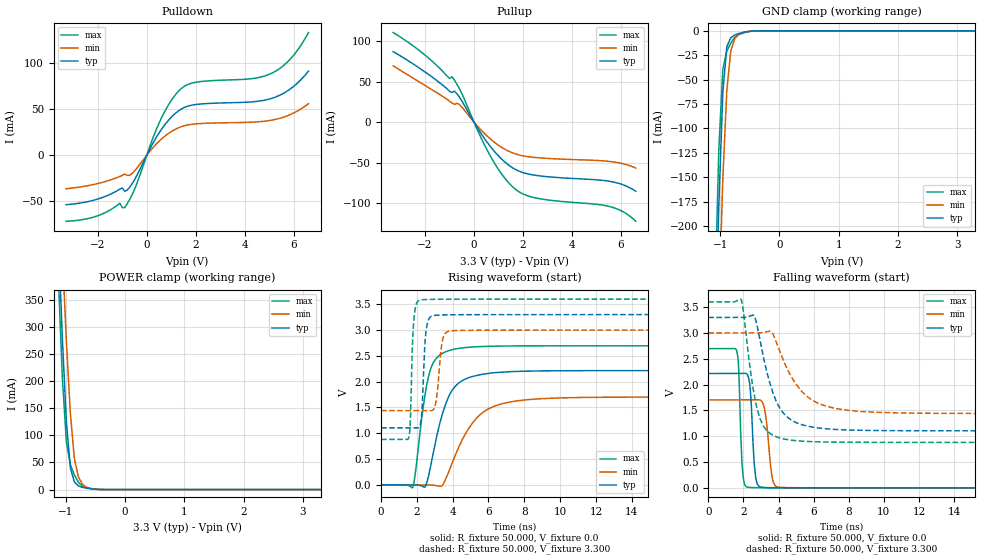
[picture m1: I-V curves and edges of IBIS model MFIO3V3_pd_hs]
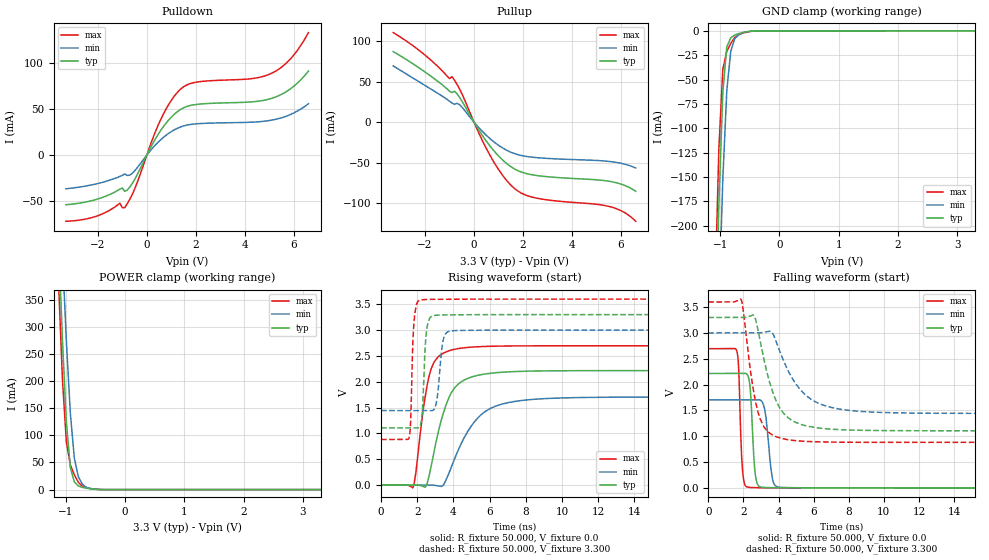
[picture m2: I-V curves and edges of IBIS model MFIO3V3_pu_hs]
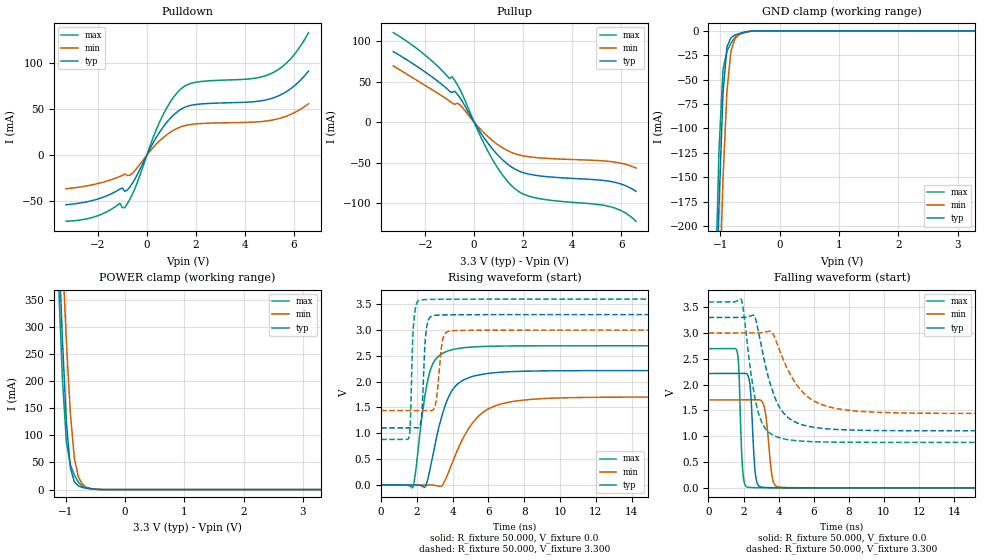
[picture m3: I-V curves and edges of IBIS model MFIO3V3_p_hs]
| IBIS file lpc55s6x_vfbga98.ibs
[IBIS Ver]   5.0
[File name]   lpc55s6x_vfbga98.ibs
[File Rev]   1.0
[Date]   May 25,2020
[Notes]   Rev History
|   1.0  initial release
[Disclaimer]   The model given below represents a 98-pin package.
[Copyright]   Copyright NXP 2020
|   Component lpc55s6x:vfbga98
[Component] lpc55s6x
[Manufacturer] NXP
[Package]
|   typ   min   max
R_pkg   0.1209   0.044925   0.28644
L_pkg   2.048e-9   9.518e-10   5.863e-9
C_pkg   3.001e-13   1.858e-13   5.678e-13
[Pin]   Signal_name   model_name   R_pin   L_pin   C_pin
G2   VDDA   POWER   NA   NA   NA
N7   USB1_3V3   POWER   NA   NA   NA
A3   USB0_3V3   POWER   NA   NA   NA
A5   VDD   POWER   NA   NA   NA
A9   VDD   POWER   NA   NA   NA
A13   VDD   POWER   NA   NA   NA
M1   VDD   POWER   NA   NA   NA
M9   VDD_PMU   POWER   NA   NA   NA
N6   USB1_DM   NC   0.094006   1.426e-9   2.165e-13
M6   USB1_DP   NC   0.094615   1.516e-9   2.317e-13
N9   FB   NC   0.12218   1.681e-9   2.209e-13
N11   LX   NC   0.06538   1.432e-9   3.1e-13
L12   P0_0   gpio3v3   0.094413   1.591e-9   2.392e-13
F5   P0_1   gpio3v3   0.09009   1.63e-9   3.407e-13
B11   P0_2   gpio3v3   0.10271   1.839e-9   2.924e-13
F8   P0_3   gpio3v3   0.1454   2.708e-9   3.901e-13
E7   P0_4   gpio3v3   0.091626   1.515e-9   3.275e-13
A7   P0_5   gpio3v3   0.12923   2.076e-9   2.188e-13
B7   P0_6   gpio3v3   0.11077   1.654e-9   2.153e-13
G5   P0_7   gpio3v3   0.13963   2.496e-9   4.691e-13
M2   P0_8   gpio3v3   0.095249   1.692e-9   2.933e-13
L13   P0_9   gpio3v3   0.15164   2.569e-9   2.247e-13
F2   P0_10   gpio3v3   0.12482   2.207e-9   3.527e-13
F1   P0_11   gpio3v3   0.13661   2.235e-9   2.226e-13
E2   P0_12   gpio3v3   0.10697   1.857e-9   3.137e-13
C12   P0_13   iicgpio3v3   0.15036   2.528e-9   2.486e-13
C13   P0_14   iicgpio3v3   0.15468   2.443e-9   2.364e-13
L2   P0_15   gpio3v3   0.098205   1.674e-9   2.761e-13
J2   P0_16   gpio3v3   0.12449   2.514e-9   2.708e-13
G3   P0_17   gpio3v3   0.075726   1.285e-9   2.687e-13
H9   P0_18   gpio3v3   0.087847   1.562e-9   3.542e-13
E6   P0_19   gpio3v3   0.083442   1.458e-9   2.858e-13
B12   P0_20   gpio3v3   0.14629   2.14e-9   2.464e-13
A12   P0_21   gpio3v3   0.12809   1.906e-9   1.918e-13
E9   P0_22   gpio3v3   0.094505   1.588e-9   3.718e-13
J1   P0_23   gpio3v3   0.13195   1.94e-9   2.141e-13
E12   P0_24   gpio3v3   0.091918   1.666e-9   2.453e-13
A11   P0_25   gpio3v3   0.11529   1.718e-9   1.949e-13
H12   P0_26   gpio3v3   0.081253   1.5e-9   2.767e-13
N2   P0_27   gpio3v3   0.13095   2.225e-9   3.428e-13
F13   P0_28   gpio3v3   0.13767   2.192e-9   2.158e-13
H8   P0_29   gpio3v3   0.15886   3.15e-9   5.678e-13
E5   P0_30   gpio3v3   0.086667   1.519e-9   3.383e-13
L1   P0_31   gpio3v3   0.15272   2.424e-9   2.59e-13
E1   P1_0   gpio3v3   0.14644   2.463e-9   2.597e-13
G11   P1_1   gpio3v3   0.096065   1.69e-9   3.188e-13
G12   P1_2   gpio3v3   0.12798   2.099e-9   2.352e-13
G13   P1_3   gpio3v3   0.12828   1.937e-9   2.153e-13
B2   P1_4   gpio3v3   0.096863   1.598e-9   2.988e-13
M5   P1_5   gpio3v3   0.094289   1.603e-9   3.053e-13
H5   P1_6   gpio3v3   0.16673   3.191e-9   4.881e-13
J5   P1_7   gpio3v3   0.12619   2.354e-9   3.979e-13
A6   P1_8   gpio3v3   0.28644   5.863e-9   4.62e-13
C1   P1_9   gpio3v3   0.1694   3.073e-9   3.031e-13
J7   P1_10   gpio3v3   0.08793   1.355e-9   3.087e-13
G6   P1_11   gpio3v3   0.15151   2.536e-9   5.272e-13
F12   P1_12   gpio3v3   0.082887   1.462e-9   2.268e-13
B3   P1_13   gpio3v3   0.11404   1.893e-9   2.97e-13
L7   P1_14   gpio3v3   0.18217   3.548e-9   3.635e-13
B6   P1_15   gpio3v3   0.12901   2.443e-9   3.381e-13
C7   P1_16   gpio3v3   0.072915   1.186e-9   2.322e-13
J9   P1_17   gpio3v3   0.10787   1.748e-9   3.803e-13
G9   P1_18   gpio3v3   0.091968   1.458e-9   3.094e-13
H13   P1_19   gpio3v3   0.12429   2.047e-9   2.027e-13
C2   P1_20   gpio3v3   0.096736   1.471e-9   2.029e-13
M7   P1_21   gpio3v3   0.14632   2.946e-9   3.43e-13
M8   P1_22   gpio3v3   0.076897   1.014e-9   2.527e-13
J8   P1_23   gpio3v3   0.085096   1.345e-9   3.077e-13
F6   P1_24   gpio3v3   0.13441   2.357e-9   4.172e-13
B8   P1_25   gpio3v3   0.10461   2.067e-9   3.287e-13
E13   P1_26   gpio3v3   0.12992   1.953e-9   2.102e-13
E8   P1_27   gpio3v3   0.11191   1.807e-9   3.572e-13
A8   P1_28   gpio3v3   0.21716   4.383e-9   3.836e-13
G8   P1_29   gpio3v3   0.15479   2.956e-9   4.522e-13
F9   P1_30   gpio3v3   0.093936   1.556e-9   3.54e-13
H6   P1_31   gpio3v3   0.14695   2.973e-9   5.442e-13
J6   RESETN   gpio3v3   0.08999   1.312e-9   3.328e-13
A1   USB0_DM   NC   0.17463   2.687e-9   2.917e-13
A2   USB0_DP   NC   0.16587   2.364e-9   2.831e-13
N13   VBAT_DCDC   NC   0.044925   1.39e-9   3.067e-13
M13   VBAT_PMU   NC   0.11627   1.679e-9   2.076e-13
N8   VBUS   NC   0.076519   9.518e-10   1.858e-13
H1   VREFN   NC   0.12485   1.889e-9   2.171e-13
G1   VREFP   NC   0.12475   1.856e-9   2.204e-13
J12   XTAL32K_N   NC   0.11411   1.691e-9   2.046e-13
J13   XTAL32K_P   NC   0.13248   1.96e-9   2.273e-13
M3   XTAL32M_N   NC   0.15178   2.164e-9   3.058e-13
N3   XTAL32M_P   NC   0.14758   1.994e-9   3.19e-13
B5   VSS   GND   NA   NA   NA
B9   VSS   GND   NA   NA   NA
B13   VSS   GND   NA   NA   NA
N1   VSS   GND   NA   NA   NA
H2   VSSA   GND   NA   NA   NA
N5   USB1_VSS   GND   NA   NA   NA
N12   VSS_DCDC   GND   NA   NA   NA
M12   VSS_DCDC   GND   NA   NA   NA
M11   VSS_PMU   GND   NA   NA   NA
B1   USB0_VSS   GND   NA   NA   NA
|   Model Selector
[Model Selector] gpio3v3
MFIO3V3_pd_hs  EPUN=1 EPD=1 EHS=1
MFIO3V3_pd_ls  EPUN=1 EPD=1 EHS=0
MFIO3V3_pu_hs  EPUN=0 EPD=0 EHS=1
MFIO3V3_pu_ls  EPUN=0 EPD=0 EHS=0
MFIO3V3_p_hs  EPUN=1 EPD=0 EHS=1
MFIO3V3_p_ls  EPUN=1 EPD=0 EHS=0
MFIO3V3_r_hs  EPUN=0 EPD=1 EHS=1
MFIO3V3_r_ls  EPUN=0 EPD=1 EHS=0
[Model Selector] iicgpio3v3
IIC3V3_pd_hs  EGP=1 EPUN=1 EPD=1 EHS=1
IIC3V3_pd_ls  EGP=1 EPUN=1 EPD=1 EHS=0
IIC3V3_p_hs  EGP=1 EPUN=1 EPD=0 EHS=1
IIC3V3_p_ls  EGP=1 EPUN=1 EPD=0 EHS=0
IIC3V3_pu_hs  EGP=1 EPUN=0 EPD=0 EHS=1
IIC3V3_pu_ls  EGP=1 EPUN=0 EPD=0 EHS=0
IIC3V3_r_hs  EGP=1 EPUN=0 EPD=1 EHS=1
IIC3V3_r_ls  EGP=1 EPUN=0 EPD=1 EHS=0
IIC3V3_pd_iic_hs  EGP=0 ECS=0 EPUN=1 EPD=1
IIC3V3_p_iic_hs  EGP=0 ECS=0 EPUN=1 EPD=0
IIC3V3_pu_iic_hs  EGP=0 ECS=0 EPUN=0 EPD=0
IIC3V3_r_iic_hs  EGP=0 ECS=0 EPUN=0 EPD=1
IIC3V3_pd_iic_pu_hs  EGP=0 ECS=1 EPUN=1 EPD=1  SSEL=1
IIC3V3_p_iic_pu_hs  EGP=0 ECS=1 EPUN=1 EPD=0  SSEL=1
IIC3V3_pu_iic_pu_hs  EGP=0 ECS=1 EPUN=0 EPD=0  SSEL=1
IIC3V3_r_iic_pu_hs  EGP=0 ECS=1 EPUN=0 EPD=1  SSEL=1
| Models and submodels in the file (24): MFIO3V3_pd_hs (I/O), MFIO3V3_pd_ls (I/O), MFIO3V3_pu_hs (I/O), MFIO3V3_pu_ls (I/O), MFIO3V3_p_hs (I/O), MFIO3V3_p_ls (I/O), MFIO3V3_r_hs (I/O), MFIO3V3_r_ls (I/O), IIC3V3_pd_hs (I/O), IIC3V3_pd_ls (I/O), IIC3V3_p_hs (I/O), IIC3V3_p_ls (I/O), IIC3V3_pu_hs (I/O), IIC3V3_pu_ls (I/O), IIC3V3_r_hs (I/O), IIC3V3_r_ls (I/O), IIC3V3_pd_iic_hs (I/O_open_drain), IIC3V3_p_iic_hs (I/O_open_drain), IIC3V3_pu_iic_hs (I/O_open_drain), IIC3V3_r_iic_hs (I/O_open_drain), IIC3V3_pd_iic_pu_hs (I/O_open_drain), IIC3V3_p_iic_pu_hs (I/O_open_drain), IIC3V3_pu_iic_pu_hs (I/O_open_drain), IIC3V3_r_iic_pu_hs (I/O_open_drain)
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|   Model MFIO3V3_pd_hs
[Model] MFIO3V3_pd_hs
Model_type I/O
Polarity   Non-Inverting
Enable   Active-Low
Vinl =  0.990V
Vinh =  2.310V
Vmeas =  1.650V
Cref =  0.0F
Rref =  100.000
Vref =  0.0V
C_comp   1.925pF   1.906pF   1.947pF
C_comp_pullup   1.145pF   1.141pF   1.152pF
C_comp_pulldown   0.641pF   0.633pF   0.647pF
[Model Spec]
Vinh   2.310V   2.100V   2.520V
Vinl   0.990V   0.900V   1.080V
Vmeas   1.650V   1.500V   1.800V
Vref   0.0V   0.0V   0.0V
Cref   0.0F   0.0F   0.0F
Rref   100.000   100.000   100.000
[Temperature Range]   25.000   0.125k   -40.000
[Voltage Range]   3.300V   3.000V   3.600V
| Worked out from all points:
|   slope of the pulldown table from 0 to 0.495 V, typ, clamps not added: 20.7 ohm
|   slope of the pullup table from 0 to 0.495 V, typ, clamps not added: 21.4 ohm
|   GND clamp passes 1 mA (typ) near -0.56 V on its own axis
|   POWER clamp passes 1 mA (typ) near -0.53 V on its own axis
|   rising waveform, R_fixture 50.000, V_fixture 0.0: 20-80 % time 1.05ns typ, 1.66ns min, 670ps max; typ from 0 V to 2.21 V
|   rising waveform, R_fixture 50.000, V_fixture 3.300: 20-80 % time 177ps typ, 247ps min, 146ps max; typ from 1.1 V to 3.3 V
|   falling waveform, R_fixture 50.000, V_fixture 0.0: 20-80 % time 203ps typ, 293ps min, 162ps max; typ from 2.21 V to 0 V
|   falling waveform, R_fixture 50.000, V_fixture 3.300: 20-80 % time 1.13ns typ, 1.67ns min, 744ps max; typ from 3.3 V to 1.1 V
[Pulldown]
|Voltage   I(typ)   I(min)   I(max)
-3.3V     -53.7mA    -36.43mA   -71.67mA
-2.1V     -48.29mA   -31.37mA   -66.51mA
-1.1V     -36.82mA   -23.05mA   -52.1mA
-900mV    -39.2mA    -20.39mA   -56.91mA
-600mV    -30.96mA   -19.83mA   -42.97mA
600mV     28.07mA    17.5mA     40.4mA
1V        41.17mA    25.53mA    59.41mA
1.4V      49.87mA    30.79mA    72.04mA
2V        54.93mA    33.94mA    79.03mA
5V        60.84mA    37.53mA    87.68mA
5.9V      72.62mA    44.52mA    105.4mA
6.6V      91.19mA    55.78mA    132.9mA
[Pullup]
|Voltage   I(typ)   I(min)   I(max)
-3.3V     87.16mA    69.54mA    110.7mA
-2.1V     64.12mA    47.22mA    85.31mA
-1V       38.1mA     25.85mA    53.88mA
-900mV    36.64mA    23.75mA    56.16mA
-800mV    38.25mA    22.02mA    51.93mA
-600mV    31.06mA    21.93mA    41.58mA
700mV     -31.25mA   -21.55mA   -43.56mA
1.2V      -47.6mA    -32.42mA   -66.97mA
1.7V      -58.52mA   -39.3mA    -83.05mA
2.6V      -66.01mA   -43.88mA   -94.06mA
5.6V      -73.4mA    -48.74mA   -104.7mA
6.6V      -85.32mA   -56.6mA    -122.4mA
[GND_clamp]
|Voltage   I(typ)   I(min)   I(max)
-3.3V     -7.222A    -7.177A    -7.278A
-1.089V   -337.1mA   -440.8mA   -274.1mA
-1.022V   -178.2mA   -284.2mA   -121mA
-955mV    -63.05mA   -151.6mA   -39.25mA
-888mV    -16.33mA   -61.34mA   -20.9mA
-821mV    -7.066mA   -20.84mA   -12.66mA
-754mV    -4.265mA   -8.157mA   -6.693mA
-687mV    -2.794mA   -3.896mA   -3.841mA
-620mV    -1.725mA   -1.894mA   -2.339mA
-419mV    -112.4uA   -138.2uA   -135uA
3.3V      0A         0A         0A
[POWER_clamp]
|Voltage   I(typ)   I(min)   I(max)
-3.3V     8.016A     7.986A     8.074A
-1.122V   463.8mA    614.4mA    385mA
-1.055V   276.3mA    435mA      203.9mA
-988mV    124.1mA    272.4mA    87.22mA
-921mV    40.03mA    140.2mA    45.68mA
-854mV    14.24mA    57.83mA    27.12mA
-787mV    6.921mA    23.8mA     13.77mA
-720mV    4.141mA    10.27mA    6.207mA
-653mV    2.682mA    4.42mA     3.699mA
-586mV    1.616mA    1.919mA    2.191mA
-452mV    346.9uA    411.9uA    422.9uA
3.3V      0A         0A         0A
[Ramp]
| variable   typ   min   max
dV/dt_r   1.328/1.048n   1.022/1.659n   1.617/0.670n
dV/dt_f   1.317/1.132n   0.935/1.671n   1.631/0.743n
R_load = 50.000
[Rising Waveform]
R_fixture= 50.000
V_fixture= 0.0
V_fixture_min= 0.0
V_fixture_max= 0.0
|time   V(typ)   V(min)   V(max)
0s        11.38nV    124.8nV    46.5nV
1.76ns    11.77uV    -454.5nV   -52.39mV
2.47ns    -34.09mV   72.05uV    1.767V
2.93ns    642.6mV    -5.154mV   2.378V
3.41ns    1.355V     -14.68mV   2.545V
3.75ns    1.693V     224.8mV    2.598V
4.9ns     2.078V     1.096V     2.667V
6.67ns    2.183V     1.564V     2.69V
10.95ns   2.213V     1.693V     2.695V
100ns     2.214V     1.703V     2.695V
[Rising Waveform]
R_fixture= 50.000
V_fixture= 3.300
V_fixture_min= 3.000
V_fixture_max= 3.600
|time   V(typ)   V(min)   V(max)
0s        1.105V     1.44V      880.4mV
1.55ns    1.105V     1.44V      919.2mV
1.84ns    1.105V     1.44V      3.234V
2.2ns     1.188V     1.44V      3.582V
2.35ns    1.923V     1.44V      3.589V
2.67ns    3.216V     1.439V     3.594V
3.06ns    3.287V     1.596V     3.596V
3.49ns    3.293V     2.878V     3.597V
4.12ns    3.296V     2.99V      3.598V
100ns     3.299V     2.999V     3.599V
[Falling Waveform]
R_fixture= 50.000
V_fixture= 0.0
V_fixture_min= 0.0
V_fixture_max= 0.0
|time   V(typ)   V(min)   V(max)
0s        2.214V     1.703V     2.695V
1.63ns    2.214V     1.703V     2.64V
1.73ns    2.214V     1.703V     2.3V
1.97ns    2.214V     1.703V     263mV
2.38ns    1.941V     1.702V     7.184mV
2.7ns     199.7mV    1.703V     3.012mV
3.2ns     7.193mV    1.543V     1.541mV
3.67ns    2.766mV    149.1mV    968.7uV
4.23ns    1.498mV    7.536mV    571.2uV
100ns     15.88nV    132.9nV    49.27nV
[Falling Waveform]
R_fixture= 50.000
V_fixture= 3.300
V_fixture_min= 3.000
V_fixture_max= 3.600
|time   V(typ)   V(min)   V(max)
0s        3.299V     2.999V     3.599V
1.87ns    3.299V     2.999V     3.646V
2.6ns     3.336V     2.999V     1.836V
3.1ns     2.603V     3.008V     1.222V
3.57ns    1.958V     3.025V     1.042V
3.85ns    1.693V     2.847V     992.4mV
5.16ns    1.242V     1.936V     908.2mV
7ns       1.136V     1.557V     885.7mV
10.97ns   1.107V     1.45V      880.6mV
100ns     1.105V     1.44V      880.4mV
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|   Model MFIO3V3_pu_hs
[Model] MFIO3V3_pu_hs
Model_type I/O
Polarity   Non-Inverting
Enable   Active-Low
Vinl =  0.990V
Vinh =  2.310V
Vmeas =  1.650V
Cref =  0.0F
Rref =  100.000
Vref =  0.0V
C_comp   1.925pF   1.906pF   1.947pF
C_comp_pullup   1.144pF   1.139pF   1.151pF
C_comp_pulldown   0.643pF   0.635pF   0.649pF
[Model Spec]
Vinh   2.310V   2.100V   2.520V
Vinl   0.990V   0.900V   1.080V
Vmeas   1.650V   1.500V   1.800V
Vref   0.0V   0.0V   0.0V
Cref   0.0F   0.0F   0.0F
Rref   100.000   100.000   100.000
[Temperature Range]   25.000   0.125k   -40.000
[Voltage Range]   3.300V   3.000V   3.600V
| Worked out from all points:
|   slope of the pulldown table from 0 to 0.495 V, typ, clamps not added: 20.7 ohm
|   slope of the pullup table from 0 to 0.495 V, typ, clamps not added: 21.4 ohm
|   GND clamp passes 1 mA (typ) near -0.55 V on its own axis
|   POWER clamp passes 1 mA (typ) near -0.54 V on its own axis
|   rising waveform, R_fixture 50.000, V_fixture 0.0: 20-80 % time 1.05ns typ, 1.65ns min, 674ps max; typ from 0.001 V to 2.21 V
|   rising waveform, R_fixture 50.000, V_fixture 3.300: 20-80 % time 179ps typ, 249ps min, 146ps max; typ from 1.11 V to 3.3 V
|   falling waveform, R_fixture 50.000, V_fixture 0.0: 20-80 % time 203ps typ, 292ps min, 162ps max; typ from 2.21 V to 0.001 V
|   falling waveform, R_fixture 50.000, V_fixture 3.300: 20-80 % time 1.14ns typ, 1.67ns min, 741ps max; typ from 3.3 V to 1.11 V
[Pulldown]
|Voltage   I(typ)   I(min)   I(max)
-3.3V     -53.7mA    -36.43mA   -71.67mA
-2.1V     -48.29mA   -31.37mA   -66.51mA
-1.1V     -36.82mA   -23.05mA   -52.1mA
-900mV    -39.2mA    -20.39mA   -56.91mA
-600mV    -30.96mA   -19.83mA   -42.97mA
600mV     28.07mA    17.5mA     40.4mA
1V        41.17mA    25.53mA    59.41mA
1.4V      49.87mA    30.79mA    72.04mA
2V        54.93mA    33.94mA    79.03mA
5V        60.84mA    37.53mA    87.68mA
5.9V      72.62mA    44.52mA    105.4mA
6.6V      91.19mA    55.78mA    132.9mA
[Pullup]
|Voltage   I(typ)   I(min)   I(max)
-3.3V     87.16mA    69.54mA    110.7mA
-2.1V     64.12mA    47.22mA    85.31mA
-1V       38.1mA     25.85mA    53.88mA
-900mV    36.64mA    23.75mA    56.16mA
-800mV    38.25mA    22.02mA    51.93mA
-600mV    31.06mA    21.93mA    41.58mA
700mV     -31.25mA   -21.55mA   -43.56mA
1.2V      -47.6mA    -32.42mA   -66.97mA
1.7V      -58.52mA   -39.3mA    -83.05mA
2.6V      -66.01mA   -43.88mA   -94.06mA
5.6V      -73.4mA    -48.74mA   -104.7mA
6.6V      -85.32mA   -56.6mA    -122.4mA
[GND_clamp]
|Voltage   I(typ)   I(min)   I(max)
-3.3V     -7.222A    -7.177A    -7.278A
-1.089V   -337.2mA   -440.9mA   -274.2mA
-1.022V   -178.3mA   -284.2mA   -121.1mA
-955mV    -63.12mA   -151.7mA   -39.33mA
-888mV    -16.39mA   -61.39mA   -20.98mA
-821mV    -7.132mA   -20.89mA   -12.74mA
-754mV    -4.331mA   -8.209mA   -6.777mA
-687mV    -2.86mA    -3.948mA   -3.925mA
-620mV    -1.791mA   -1.946mA   -2.423mA
-419mV    -178.1uA   -190.3uA   -219.1uA
3.3V      0A         0A         0A
[POWER_clamp]
|Voltage   I(typ)   I(min)   I(max)
-3.3V     8.016A     7.986A     8.074A
-1.122V   463.7mA    614.3mA    385mA
-1.055V   276.3mA    434.9mA    203.9mA
-988mV    124mA      272.3mA    87.13mA
-921mV    39.96mA    140.1mA    45.6mA
-854mV    14.17mA    57.77mA    27.03mA
-787mV    6.855mA    23.75mA    13.68mA
-720mV    4.075mA    10.22mA    6.123mA
-653mV    2.616mA    4.368mA    3.615mA
-586mV    1.55mA     1.867mA    2.107mA
-452mV    281.1uA    359.9uA    338.7uA
3.3V      0A         0A         0A
[Ramp]
| variable   typ   min   max
dV/dt_r   1.329/1.048n   1.022/1.658n   1.617/0.670n
dV/dt_f   1.316/1.133n   0.935/1.672n   1.631/0.744n
R_load = 50.000
[Rising Waveform]
R_fixture= 50.000
V_fixture= 0.0
V_fixture_min= 0.0
V_fixture_max= 0.0
|time   V(typ)   V(min)   V(max)
0s        869.8uV    949.2uV    842.8uV
1.76ns    883.1uV    948.7uV    -50.04mV
2.46ns    -36.02mV   1.019mV    1.752V
2.89ns    574.4mV    -2.025mV   2.352V
3.38ns    1.318V     -20.64mV   2.54V
3.71ns    1.664V     197mV      2.595V
4.93ns    2.083V     1.116V     2.669V
6.71ns    2.185V     1.57V      2.691V
10.86ns   2.214V     1.693V     2.696V
100ns     2.215V     1.704V     2.696V
[Rising Waveform]
R_fixture= 50.000
V_fixture= 3.300
V_fixture_min= 3.000
V_fixture_max= 3.600
|time   V(typ)   V(min)   V(max)
0s        1.106V     1.442V     881.7mV
1.55ns    1.106V     1.442V     920.7mV
1.83ns    1.106V     1.442V     3.201V
2.2ns     1.19V      1.442V     3.584V
2.36ns    2.014V     1.442V     3.591V
2.67ns    3.219V     1.441V     3.595V
3.07ns    3.288V     1.618V     3.597V
3.47ns    3.295V     2.857V     3.598V
4.1ns     3.297V     2.991V     3.599V
100ns     3.3V       3V         3.6V
[Falling Waveform]
R_fixture= 50.000
V_fixture= 0.0
V_fixture_min= 0.0
V_fixture_max= 0.0
|time   V(typ)   V(min)   V(max)
0s        2.215V     1.704V     2.696V
1.63ns    2.215V     1.704V     2.641V
1.73ns    2.215V     1.704V     2.3V
1.97ns    2.216V     1.704V     265.9mV
2.37ns    1.988V     1.704V     8.752mV
2.68ns    252.6mV    1.704V     4.211mV
3.22ns    8.138mV    1.504V     2.448mV
3.66ns    3.888mV    167.2mV    1.863mV
4.25ns    2.441mV    8.626mV    1.426mV
100ns     869.8uV    949.3uV    842.8uV
[Falling Waveform]
R_fixture= 50.000
V_fixture= 3.300
V_fixture_min= 3.000
V_fixture_max= 3.600
|time   V(typ)   V(min)   V(max)
0s        3.3V       3V         3.6V
1.87ns    3.3V       3V         3.648V
2.61ns    3.334V     3V         1.81V
3.09ns    2.622V     3.009V     1.234V
3.58ns    1.952V     3.025V     1.042V
3.83ns    1.711V     2.861V     997mV
5.1ns     1.252V     1.964V     911.3mV
6.89ns    1.14V      1.568V     887.6mV
10.88ns   1.108V     1.453V     881.9mV
100ns     1.106V     1.442V     881.7mV
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|   Model MFIO3V3_p_hs
[Model] MFIO3V3_p_hs
Model_type I/O
Polarity   Non-Inverting
Enable   Active-Low
Vinl =  0.990V
Vinh =  2.310V
Vmeas =  1.650V
Cref =  0.0F
Rref =  100.000
Vref =  0.0V
C_comp   1.925pF   1.906pF   1.947pF
C_comp_pullup   1.144pF   1.140pF   1.152pF
C_comp_pulldown   0.642pF   0.634pF   0.649pF
[Model Spec]
Vinh   2.310V   2.100V   2.520V
Vinl   0.990V   0.900V   1.080V
Vmeas   1.650V   1.500V   1.800V
Vref   0.0V   0.0V   0.0V
Cref   0.0F   0.0F   0.0F
Rref   100.000   100.000   100.000
[Temperature Range]   25.000   0.125k   -40.000
[Voltage Range]   3.300V   3.000V   3.600V
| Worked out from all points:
|   slope of the pulldown table from 0 to 0.495 V, typ, clamps not added: 20.7 ohm
|   slope of the pullup table from 0 to 0.495 V, typ, clamps not added: 21.4 ohm
|   GND clamp passes 1 mA (typ) near -0.56 V on its own axis
|   POWER clamp passes 1 mA (typ) near -0.54 V on its own axis
|   rising waveform, R_fixture 50.000, V_fixture 0.0: 20-80 % time 1.05ns typ, 1.66ns min, 670ps max; typ from 0 V to 2.21 V
|   rising waveform, R_fixture 50.000, V_fixture 3.300: 20-80 % time 177ps typ, 254ps min, 147ps max; typ from 1.1 V to 3.3 V
|   falling waveform, R_fixture 50.000, V_fixture 0.0: 20-80 % time 203ps typ, 291ps min, 162ps max; typ from 2.21 V to 0 V
|   falling waveform, R_fixture 50.000, V_fixture 3.300: 20-80 % time 1.14ns typ, 1.68ns min, 740ps max; typ from 3.3 V to 1.1 V
[Pulldown]
|Voltage   I(typ)   I(min)   I(max)
-3.3V     -53.7mA    -36.43mA   -71.67mA
-2.1V     -48.29mA   -31.37mA   -66.51mA
-1.1V     -36.82mA   -23.05mA   -52.1mA
-900mV    -39.2mA    -20.39mA   -56.91mA
-600mV    -30.96mA   -19.83mA   -42.97mA
600mV     28.07mA    17.5mA     40.4mA
1V        41.17mA    25.53mA    59.41mA
1.4V      49.87mA    30.79mA    72.04mA
2V        54.93mA    33.94mA    79.03mA
5V        60.84mA    37.53mA    87.68mA
5.9V      72.62mA    44.52mA    105.4mA
6.6V      91.19mA    55.78mA    132.9mA
[Pullup]
|Voltage   I(typ)   I(min)   I(max)
-3.3V     87.16mA    69.54mA    110.7mA
-2.1V     64.12mA    47.22mA    85.31mA
-1V       38.1mA     25.85mA    53.88mA
-900mV    36.64mA    23.75mA    56.16mA
-800mV    38.25mA    22.02mA    51.93mA
-600mV    31.06mA    21.93mA    41.58mA
700mV     -31.25mA   -21.55mA   -43.56mA
1.2V      -47.6mA    -32.42mA   -66.97mA
1.7V      -58.52mA   -39.3mA    -83.05mA
2.6V      -66.01mA   -43.88mA   -94.06mA
5.6V      -73.4mA    -48.74mA   -104.7mA
6.6V      -85.32mA   -56.6mA    -122.4mA
[GND_clamp]
|Voltage   I(typ)   I(min)   I(max)
-3.3V     -7.222A    -7.177A    -7.278A
-1.089V   -337.1mA   -440.8mA   -274.1mA
-1.022V   -178.2mA   -284.2mA   -121mA
-955mV    -63.04mA   -151.6mA   -39.24mA
-888mV    -16.32mA   -61.33mA   -20.89mA
-821mV    -7.057mA   -20.83mA   -12.64mA
-754mV    -4.256mA   -8.15mA    -6.682mA
-687mV    -2.785mA   -3.888mA   -3.83mA
-620mV    -1.717mA   -1.887mA   -2.329mA
-419mV    -104.8uA   -131.8uA   -126uA
3.3V      0A         0A         0A
[POWER_clamp]
|Voltage   I(typ)   I(min)   I(max)
-3.3V     8.016A     7.986A     8.074A
-1.122V   463.7mA    614.3mA    384.9mA
-1.055V   276.2mA    434.9mA    203.8mA
-988mV    124mA      272.3mA    87.12mA
-921mV    39.95mA    140.1mA    45.59mA
-854mV    14.16mA    57.77mA    27.02mA
-787mV    6.846mA    23.74mA    13.67mA
-720mV    4.066mA    10.21mA    6.113mA
-653mV    2.607mA    4.361mA    3.605mA
-586mV    1.542mA    1.86mA     2.097mA
-452mV    273.4uA    353.7uA    329.6uA
3.3V      0A         0A         0A
[Ramp]
| variable   typ   min   max
dV/dt_r   1.329/1.049n   1.022/1.660n   1.618/0.670n
dV/dt_f   1.317/1.134n   0.935/1.674n   1.632/0.744n
R_load = 50.000
[Rising Waveform]
R_fixture= 50.000
V_fixture= 0.0
V_fixture_min= 0.0
V_fixture_max= 0.0
|time   V(typ)   V(min)   V(max)
0s        11.91nV    127.2nV    48.18nV
1.76ns    14.07uV    -452.3nV   -52.48mV
1.9ns     130.3uV    -183.4nV   185.6mV
2.46ns    -38.99mV   68.8uV     1.761V
2.93ns    644.9mV    -5.155mV   2.378V
3.65ns    1.606V     144.1mV    2.586V
4.94ns    2.084V     1.117V     2.669V
6.67ns    2.183V     1.565V     2.691V
10.87ns   2.214V     1.693V     2.696V
100ns     2.215V     1.703V     2.696V
[Rising Waveform]
R_fixture= 50.000
V_fixture= 3.300
V_fixture_min= 3.000
V_fixture_max= 3.600
|time   V(typ)   V(min)   V(max)
0s        1.105V     1.441V     880.7mV
1.55ns    1.105V     1.441V     919.6mV
1.84ns    1.105V     1.441V     3.233V
2.22ns    1.224V     1.441V     3.584V
2.37ns    2.139V     1.441V     3.59V
2.69ns    3.23V      1.44V      3.595V
3.05ns    3.287V     1.579V     3.596V
3.48ns    3.294V     2.867V     3.598V
4.12ns    3.297V     2.991V     3.599V
100ns     3.3V       3V         3.6V
[Falling Waveform]
R_fixture= 50.000
V_fixture= 0.0
V_fixture_min= 0.0
V_fixture_max= 0.0
|time   V(typ)   V(min)   V(max)
0s        2.215V     1.703V     2.696V
1.62ns    2.215V     1.703V     2.651V
1.73ns    2.215V     1.703V     2.303V
1.97ns    2.215V     1.703V     265.7mV
2.37ns    1.981V     1.703V     8.251mV
2.69ns    225.2mV    1.704V     3.621mV
3.22ns    7.595mV    1.504V     1.863mV
3.67ns    3.256mV    150.5mV    1.23mV
4.25ns    1.815mV    7.854mV    743.4uV
100ns     16.41nV    135.3nV    50.94nV
[Falling Waveform]
R_fixture= 50.000
V_fixture= 3.300
V_fixture_min= 3.000
V_fixture_max= 3.600
|time   V(typ)   V(min)   V(max)
0s        3.3V       3V         3.6V
1.88ns    3.3V       3V         3.641V
2.61ns    3.334V     3V         1.821V
3.08ns    2.642V     3.008V     1.24V
3.58ns    1.951V     3.025V     1.041V
3.83ns    1.711V     2.865V     995.8mV
5.17ns    1.242V     1.934V     908.5mV
7.01ns    1.137V     1.557V     886.1mV
10.99ns   1.107V     1.451V     880.9mV
100ns     1.105V     1.441V     880.7mV
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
